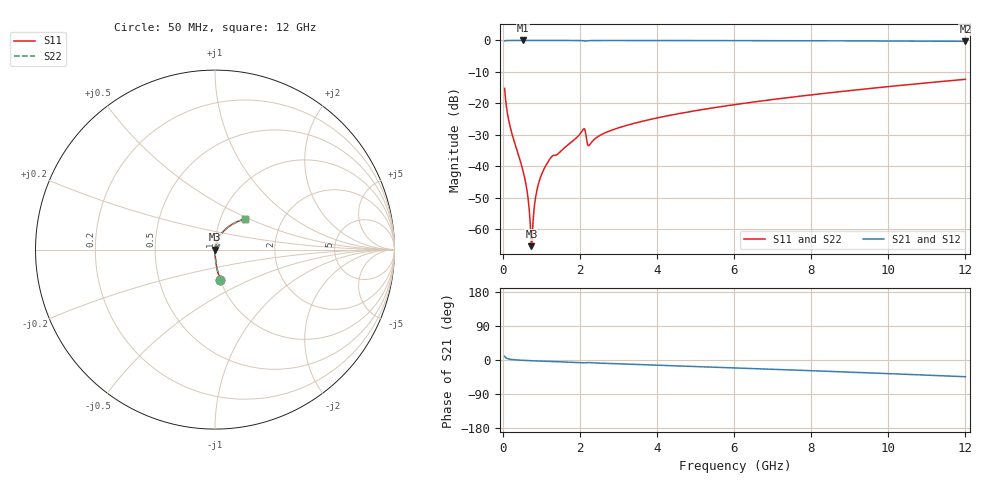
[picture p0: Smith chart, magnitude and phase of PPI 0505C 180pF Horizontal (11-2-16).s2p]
# MHz S MA R 50
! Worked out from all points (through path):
!   1601 points, 50 MHz to 12 GHz, reference 50 ohm
!   highest |S21| = 0.00 dB at 528 MHz (marker M1); lowest = -0.3 dB at 12 GHz (marker M2)
!   group delay of S21, straight-line fit = 10.4 ps
!   lowest |S11| = -65.3 dB at 744.6 MHz (marker M3), VSWR 1.00, Z = 50.1 - j0.0138 ohm
!   |S11| at or under -10 dB: start of sweep to end of sweep
!   |S22| runs from -65.3 to -12.3 dB; largest |S21 - S12| = 0
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50  0.1731 -80.1  0.9847 9.8  0.9847 9.8  0.1731 -80.1
206.8438  0.03941 -87.8  0.9989 1.7  0.9989 1.7  0.03941 -87.8
528  0.008459 -87.8  0.9995 -0.9  0.9995 -0.9  0.008459 -87.8
625.0938  0.004335 -84.9  0.9995 -1.4  0.9995 -1.4  0.004335 -84.9
707.25  0.001445 -70.9  0.9994 -1.7  0.9994 -1.7  0.001445 -70.9
744.5938  0.000541 -14.8  0.9994 -1.9  0.9994 -1.9  0.000541 -14.8
781.9375  0.001183 60.8  0.9994 -2.1  0.9994 -2.1  0.001183 60.8
849.1562  0.003102 77.2  0.9994 -2.4  0.9994 -2.4  0.003102 77.2
908.9062  0.004767 80.3  0.9993 -2.6  0.9993 -2.6  0.004767 80.3
991.0625  0.006968 81.8  0.9993 -3.0  0.9993 -3.0  0.006968 81.8
1103.094  0.00989 82.2  0.9991 -3.4  0.9991 -3.4  0.00989 82.2
1267.406  0.01421 78.8  0.9981 -4.1  0.9981 -4.1  0.01421 78.8
2044.156  0.03527 73.9  0.9938 -7.3  0.9938 -7.3  0.03527 73.9
2111.375  0.03958 59.4  0.9837 -7.5  0.9837 -7.5  0.03958 59.4
2208.469  0.02173 53.1  0.9888 -6.8  0.9888 -6.8  0.02173 53.1
2253.281  0.0219 67.0  0.9936 -7.0  0.9936 -7.0  0.0219 67.0
2776.094  0.03661 78.8  0.9979 -9.2  0.9979 -9.2  0.03661 78.8
4038.312  0.05941 75.1  0.9968 -13.8  0.9968 -13.8  0.05941 75.1
6025  0.09583 68.3  0.9937 -20.9  0.9937 -20.9  0.09583 68.3
8019.156  0.1371 61.1  0.9885 -28.3  0.9885 -28.3  0.1371 61.1
10013.31  0.1851 53.5  0.9803 -36.0  0.9803 -36.0  0.1851 53.5
12000  0.2414 45.4  0.9676 -44.1  0.9676 -44.1  0.2414 45.4
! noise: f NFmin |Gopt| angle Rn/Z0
50  0.0003255  0.8401  0.2823  0.000431
1372  0.005956  0.7694  3.506  0.005256
2701  0.006087  0.5989  6.678  0.002785
4031  0.007129  0.5163  9.572  0.002557
5360  0.008694  0.4849  12.4  0.002856
6682  0.01027  0.4652  15.11  0.00319
8012  0.01186  0.4525  17.73  0.00355
9341  0.0135  0.445  20.25  0.003941
1.067e+04  0.01521  0.4419  22.69  0.004376
1.2e+04  0.01702  0.4427  25.06  0.004868
